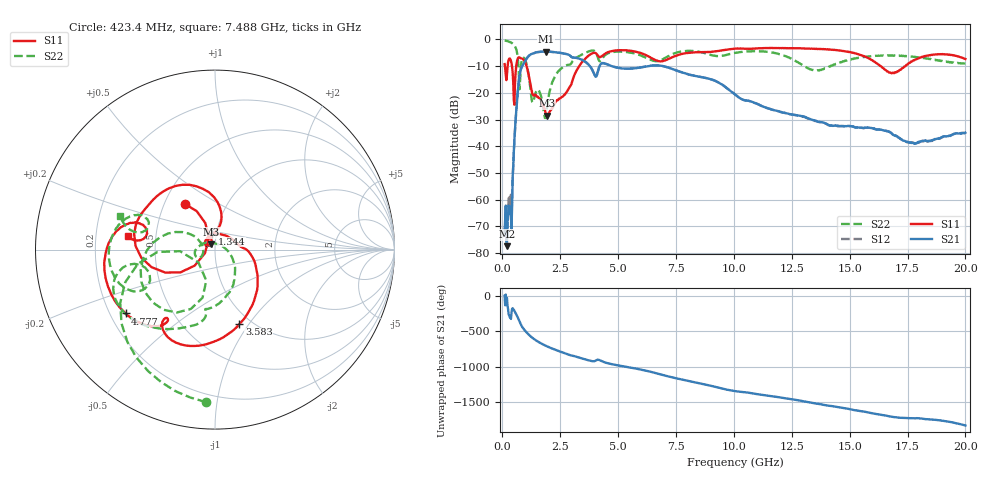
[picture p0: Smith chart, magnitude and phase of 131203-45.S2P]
!  2-Port S-parameters saved by WinCal
! VAR MeasName=S-Parameters (CALIBRATED_DATA) read from VNA (N5244A)
! VAR MeasDate=4/4/2013 3:58:55 PM
! VAR NAME=131203-45
! VAR FILENAME=131203-45.S2P
! VAR DATE=4/4/2013 3:58:55 PM
! VAR PHYS_PORTS=1,2
# Hz S MA R 50
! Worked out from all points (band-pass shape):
!   801 points, 100 MHz to 20 GHz, reference 50 ohm
!   highest |S21| = -4.52 dB at 1.891 GHz (marker M1); lowest = -77.4 dB at 199.5 MHz (marker M2)
!   |S21| within 3 dB of the highest: 1.026 GHz to 3.415 GHz (2.389 GHz wide, 108 % of centre)
!   lowest |S11| = -28.6 dB at 1.916 GHz (marker M3), VSWR 1.08, Z = 47.7 + j2.82 ohm
!   |S11| at or under -10 dB: 417.3 MHz to 602.2 MHz (184.9 MHz wide, 36.3 % of centre); 1.049 GHz to 3.317 GHz (2.268 GHz wide, 104 % of centre); 16.34 GHz to 17.41 GHz (1.068 GHz wide, 6.33 % of centre)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
!   |S22| runs from -29.4 to -0.4 dB; largest |S21 - S12| = 0.0029
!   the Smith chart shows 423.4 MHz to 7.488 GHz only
!   S11 on the Smith chart (normalised r, x): 423.4 MHz: 0.64, +0.36; 1.344 GHz: 0.95, +0.17; 3.583 GHz: 0.88, -0.90; 4.777 GHz: 0.26, -0.30; 7.488 GHz: 0.34, +0.07
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1e8  0.3455 152.9  0.0002346 -1.2  0.0002814 -34.4  0.9573 -22.2
1.995e8  0.2141 -168.0  0.0001346 -28.7  0.000288 -150.1  0.9366 -43.5
4.23375e8  0.3041 123.3  0.0007647 176.2  0.001054 -162.9  0.8508 -93.4
5.72625e8  0.2303 -146.6  0.02955 117.0  0.02948 116.9  0.7089 -133.5
7.4675e8  0.4584 155.4  0.2149 -3.8  0.2149 -3.8  0.1171 -142.0
9.70625e8  0.3869 111.2  0.3841 -125.8  0.3848 -125.8  0.4297 -164.5
1.14475e9  0.2098 80.5  0.4917 173.0  0.4931 173.1  0.2063 151.7
1.34375e9  0.09038 100.5  0.5486 117.7  0.5501 117.7  0.0699 -162.7
1.891e9  0.03832 121.8  0.594 15.2  0.5957 15.1  0.03938 36.7
1.915875e9  0.03715 127.5  0.5937 11.3  0.5951 11.3  0.0486 18.5
2.5875e9  0.08461 92.9  0.5529 -74.9  0.5538 -74.9  0.2956 -84.5
3.43325e9  0.3712 -55.7  0.4167 -160.3  0.4186 -160.2  0.5185 -121.5
3.5825e9  0.4367 -71.8  0.3818 -174.5  0.3842 -174.4  0.5582 -129.2
4.7765e9  0.6117 -144.5  0.312 115.2  0.3134 114.9  0.5818 -166.0
6.741625e9  0.3937 164.3  0.3262 -16.9  0.3272 -17.1  0.3967 163.1
7.487875e9  0.4924 171.5  0.2653 -78.2  0.2659 -78.6  0.56 160.5
1.005e10  0.672 133.7  0.09366 100.2  0.09342 99.4  0.5612 125.0
1.338325e10  0.67 85.0  0.03129 -65.2  0.03078 -65.4  0.268 84.2
1.539812e10  0.5264 49.9  0.02231 -176.4  0.02239 -176.2  0.4569 98.3
1.669162e10  0.2427 52.0  0.0186 106.5  0.01898 107.1  0.4967 80.2
1.843288e10  0.5073 65.5  0.01266 63.3  0.01247 62.9  0.4296 61.1
2e10  0.4306 22.3  0.01787 -22.6  0.01763 -23.0  0.3553 59.6
